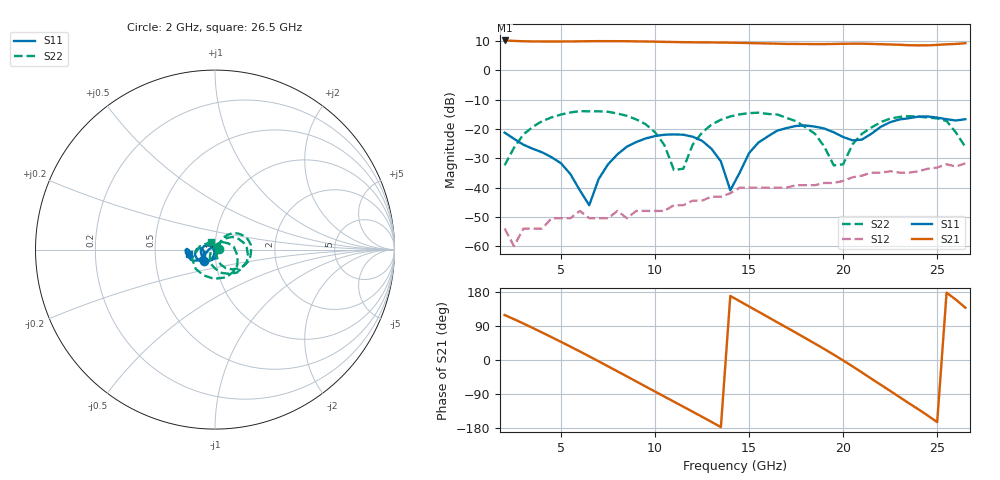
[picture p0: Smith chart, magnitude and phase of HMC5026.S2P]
! HMMC-5026
! Typical S-Parameters Ta=25 C, VDD=7V, ID=150mA or IDSS (whichever is less)
# ghz s ma r 50
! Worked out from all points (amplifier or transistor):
!   50 points, 2 GHz to 26.5 GHz, reference 50 ohm
!   highest |S21| = 10.3 dB at 2 GHz (marker M1)
!   |S21| within 3 dB of that: start of sweep to end of sweep
!   unconditionally stable (mu >= 1): start of sweep to end of sweep
!   at 6 GHz: K = 38.11, MAG = 10.1 dB, |S12| = -48.0 dB
!   at 14.5 GHz: K = 16.34, MAG = 9.6 dB, |S12| = -40.0 dB
!   at 26.5 GHz: K = 6.45, MAG = 9.4 dB, |S12| = -31.7 dB
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2  0.087 -134.8  3.255 118.6  0.002 154.9  0.024 14.4
4  0.04 -173.6  3.126 72.4  0.002 79.9  0.137 42.6
5  0.026 163.8  3.125 47.8  0.003 57.4  0.177 26.0
6.5  0.005 20.1  3.161 9.6  0.003 15.3  0.201 -1.4
8  0.037 -78.1  3.166 -29.9  0.004 -29.8  0.184 -29.6
9.5  0.069 -118.3  3.125 -70.0  0.004 -48.8  0.121 -59.6
10.5  0.08 -146.2  3.077 -96.6  0.004 -75.8  0.053 -75.8
11.5  0.08 -170.8  3.042 -123.2  0.005 -91.6  0.021 57.4
12.5  0.063 161.0  3.017 -149.9  0.006 -113.5  0.087 46.0
14  0.009 150.7  2.984 169.0  0.008 -151.8  0.164 13.4
14.5  0.018 -98.2  2.964 155.2  0.01 -160.8  0.178 2.6
16.5  0.094 -131.4  2.868 99.4  0.01 140.9  0.177 -46.5
17.5  0.113 -154.2  2.837 71.7  0.011 119.1  0.136 -73.5
18.5  0.11 -173.8  2.824 43.3  0.011 91.2  0.083 -106.1
19.5  0.088 175.2  2.836 14.0  0.012 70.6  0.024 -166.7
20.5  0.064 -174.9  2.868 -16.8  0.015 41.3  0.055 52.8
21.5  0.083 -150.6  2.84 -49.3  0.018 18.5  0.106 8.5
22.5  0.131 -151.8  2.781 -81.5  0.019 -19.5  0.151 -34.4
23.5  0.153 -164.6  2.702 -114.2  0.018 -54.6  0.166 -68.9
25  0.157 178.6  2.731 -163.9  0.022 -96.5  0.152 -134.8
26  0.14 -174.1  2.839 159.1  0.023 -138.5  0.087 168.1
26.5  0.147 -169.8  2.925 137.9  0.026 -155.0  0.049 116.0
